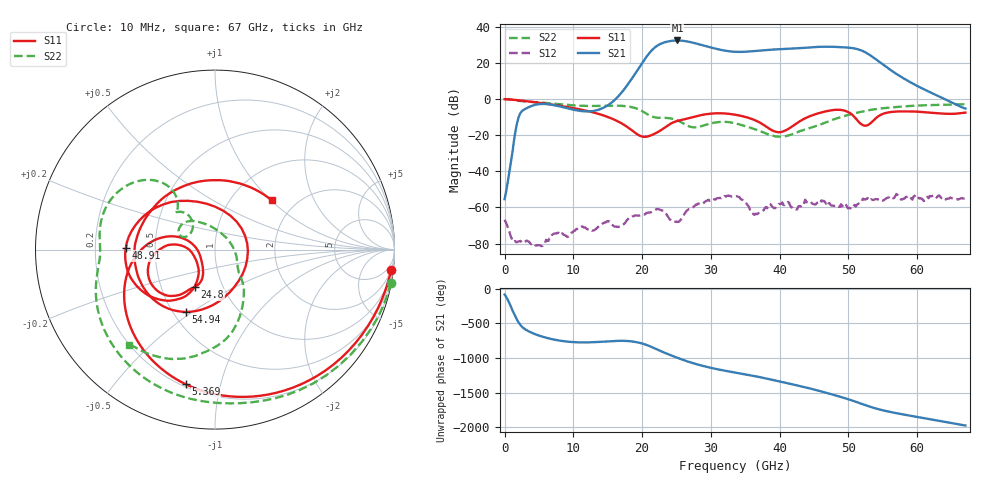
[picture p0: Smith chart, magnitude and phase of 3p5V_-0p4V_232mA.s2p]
! MARKI MICROWAVE INC.
! Date:  10/23/18
! Model Number:  AMM-6702CH
! Description:  2-port Small Signal S-parameter data for AMM-6702CH
! Frequency Range:  10 MHz to 67 GHz
! Port Configuration:  PORT 1: Input
!  PORT 2: Output
! Bias Condition: Vd = +3.5V, Vg = -0.4V
! AMM-6702CH s2p files are only valid for small signal conditions (below -5 dBm input power)
!S2P File: Measurements: Mag<S11> Ang<S11>, Mag<S21> Ang<S21>, Mag<S12> Ang<S12>, Mag<S22> Ang<S22>!row 1
# Hz S  dB  R 50
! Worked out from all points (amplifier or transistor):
!   401 points, 10 MHz to 67 GHz, reference 50 ohm
!   highest |S21| = 32.4 dB at 25.13 GHz (marker M1)
!   |S21| within 3 dB of that: 22.16 GHz to 29.13 GHz (6.971 GHz wide, 27.2 % of centre)
!   unconditionally stable (mu >= 1): start of sweep to end of sweep
!   at 11.06 GHz: K = 1574.31, MAG = -2.9 dB, |S12| = -70.7 dB
!   at 33.51 GHz: K = 10.16, MAG = 26.9 dB, |S12| = -53.9 dB
!   at 67 GHz: K = 210.92, MAG = -1.4 dB, |S12| = -55.1 dB
!   S11 on the Smith chart (normalised r, x): 10 MHz: 2, -17; 5.369 GHz: 0.21, -0.78; 24.8 GHz: 0.74, -0.33; 48.91 GHz: 0.34, +0.01; 54.94 GHz: 0.58, -0.47; 67 GHz: 1.51, +1.01
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1e7  -0.11 -6.7  -55.41 -86.3  -66.77 -30.0  -0.02 -10.8
5.3692e9  -2.29 -102.2  -2.76 31.1  -81.40 -107.9  -2.01 -131.0
1.123082e10  -5.96 -165.3  -6.72 -56.2  -70.46 166.2  -3.77 -174.2
1.993952e10  -20.72 -170.7  19.51 -70.2  -63.94 132.2  -6.55 128.0
2.14468e10  -19.86 -136.2  27.05 -124.7  -62.25 122.3  -9.74 129.5
2.245165e10  -17.92 -121.9  30.05 -169.5  -61.02 100.6  -10.45 135.8
2.34565e10  -15.43 -114.2  31.52 147.3  -63.26 65.3  -10.46 136.1
2.47963e10  -12.54 -118.2  32.32 94.7  -67.90 -80.0  -11.36 130.2
2.513125e10  -12.14 -120.2  32.36 82.0  -68.01 -120.1  -11.83 128.7
2.74759e10  -9.93 -127.9  31.04 2.9  -59.74 137.0  -15.69 143.6
2.982055e10  -8.18 -142.2  28.64 -58.4  -56.38 99.6  -13.69 158.3
3.3505e10  -8.69 -170.4  26.08 -129.4  -53.93 39.2  -13.42 132.0
3.718945e10  -13.22 172.6  26.79 162.2  -62.59 -142.4  -17.82 98.3
4.037148e10  -18.14 -143.8  27.60 93.2  -57.19 30.4  -20.85 35.0
4.472582e10  -9.04 -127.8  28.61 -7.5  -57.84 -82.8  -15.67 -39.2
4.707048e10  -6.56 -151.3  28.90 -70.1  -57.57 144.5  -12.44 -49.8
4.89127e10  -6.07 178.9  28.65 -122.4  -58.20 -55.3  -9.96 -60.0
5.058745e10  -8.85 132.8  28.12 -174.6  -59.98 150.3  -8.18 -68.9
5.209472e10  -14.45 38.8  26.47 133.0  -55.07 -77.7  -6.90 -76.3
5.49418e10  -8.34 -114.8  19.25 47.4  -56.27 -53.4  -5.15 -91.8
5.594665e10  -7.33 -133.6  16.50 24.9  -54.58 38.7  -4.79 -96.1
6.7e10  -7.57 41.1  -5.28 -172.4  -55.08 4.7  -2.93 -132.0
